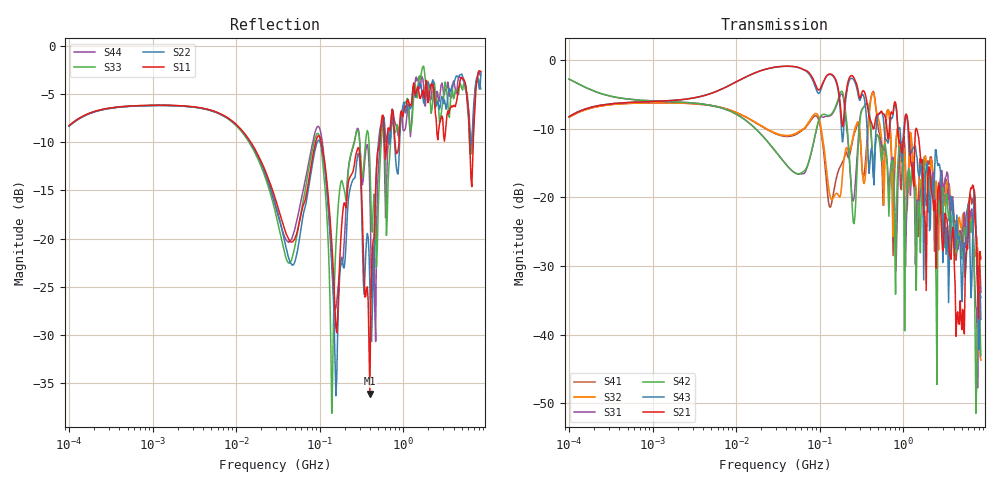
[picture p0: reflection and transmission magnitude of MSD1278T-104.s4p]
# MHz S MA R 50
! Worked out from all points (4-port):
!   498 points, 100 kHz to 8.5 GHz, reference 50 ohm
!   strongest paths, dB at 100 kHz, 1.698 MHz, 29.49 MHz, 500.7 MHz, 8.5 GHz:
!     S21: -8.3, -5.9, -1.0, -7.9, -29.0
!     S43: -8.2, -5.9, -1.0, -8.0, -34.6
!     S42: -2.8, -6.1, -13.3, -11.1, -43.1
!     S31: -2.8, -6.1, -13.3, -11.1, -37.8
!     S32: -8.4, -6.3, -10.6, -8.4, -43.7
!     S41: -8.3, -6.3, -10.7, -9.8, -33.8
!   lowest |S11| = -36.1 dB at 398.4 MHz (marker M1), VSWR 1.03, Z = 51.4 + j0.74 ohm
!   |S11| at or under -10 dB: 104 MHz to 520.7 MHz (416.7 MHz wide, 133 % of centre); 798.4 MHz to 888.4 MHz (90.06 MHz wide, 10.7 % of centre); 6.255 GHz to 6.894 GHz (639.1 MHz wide, 9.72 % of centre)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
0.1  0.3863 36.6  0.3866 37.9  0.7255 -19.2  0.3826 -143.1
     0.3866 37.9  0.3829 36.8  0.3822 -143.1  0.727 -19.2
     0.7255 -19.2  0.3822 -143.1  0.3855 36.8  0.3874 37.7
     0.3826 -143.1  0.727 -19.2  0.3874 37.7  0.3838 37.0
94.51579  0.3398 -23.2  0.6133 -29.3  0.3406 137.0  0.382 3.8
          0.6133 -29.3  0.3207 -20.6  0.3996 1.0  0.3417 139.1
          0.3406 137.0  0.3996 1.0  0.3519 -19.7  0.5784 -31.8
          0.382 3.8  0.3417 139.1  0.5784 -31.8  0.3822 -18.7
139.353  0.09485 -108.2  0.7852 -38.1  0.401 45.5  0.09201 16.7
         0.7852 -38.1  0.07726 -108.3  0.09664 -7.0  0.4077 48.9
         0.401 45.5  0.09664 -7.0  0.01239 -30.6  0.7769 -42.9
         0.09201 16.7  0.4077 48.9  0.7769 -42.9  0.07379 -67.7
398.4376  0.01567 27.3  0.3717 -85.1  0.3696 -61.0  0.4751 0.1
          0.3717 -85.1  0.05774 -39.9  0.4522 7.0  0.3824 -62.4
          0.3696 -61.0  0.4522 7.0  0.2492 -86.8  0.1735 -74.3
          0.4751 0.1  0.3824 -62.4  0.1735 -74.3  0.1759 -91.9
561.2231  0.4362 -6.4  0.4106 -89.2  0.2292 -83.1  0.1458 -96.4
          0.4106 -89.2  0.3825 -1.9  0.2222 -97.2  0.2039 -75.3
          0.2292 -83.1  0.2222 -97.2  0.3677 -3.9  0.4112 -84.3
          0.1458 -96.4  0.2039 -75.3  0.4112 -84.3  0.3755 -20.4
2972.863  0.4189 77.1  0.04072 135.5  0.1203 45.6  0.0926 60.3
          0.04072 135.5  0.5284 86.0  0.1192 57.6  0.1177 45.4
          0.1203 45.6  0.1192 57.6  0.5057 89.1  0.03345 -141.7
          0.0926 60.3  0.1177 45.4  0.03345 -141.7  0.6118 86.7
8500  0.736 -50.8  0.03564 -105.9  0.01294 -119.0  0.02032 -141.5
      0.03564 -105.9  0.7251 -39.2  0.006502 22.1  0.007009 -55.9
      0.01294 -119.0  0.006502 22.1  0.5994 -42.7  0.01859 -70.4
      0.02032 -141.5  0.007009 -55.9  0.01859 -70.4  0.7082 -46.5
